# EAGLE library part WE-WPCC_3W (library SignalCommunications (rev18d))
WE-WPCC Wireless Power Charging Coil Characteristics Qi-standard compliant Evaluated and approved by every major semiconductor manufacturer Litzwire used – highest Q-value available on market Applicable for up to 20 W High permeability shielding Cancels charging flux to be not coupled into sensitive components or batteries High reliable construction Applications Portable devices used in a clean area, where connectors pose a risk of polluting e.g. medical facilities, (industrial) clean rooms, mining industry Devices with a large number of mating cycles to avoid connector damage: eg. Smart watches, fitness tracker … Consumer products: eg. Digital cameras, baby phone, walkie talky, remote control, smartphone sleeves, watertight products Explosion sensitive area where the use of a physical connection is hazardous Smart sensors Details see: http://katalog.we-online.de/en/pbs/WE-WPCC-ARRAY Created by Dan Xu 2014-05-21 2014 (C) Wurth Elektronik
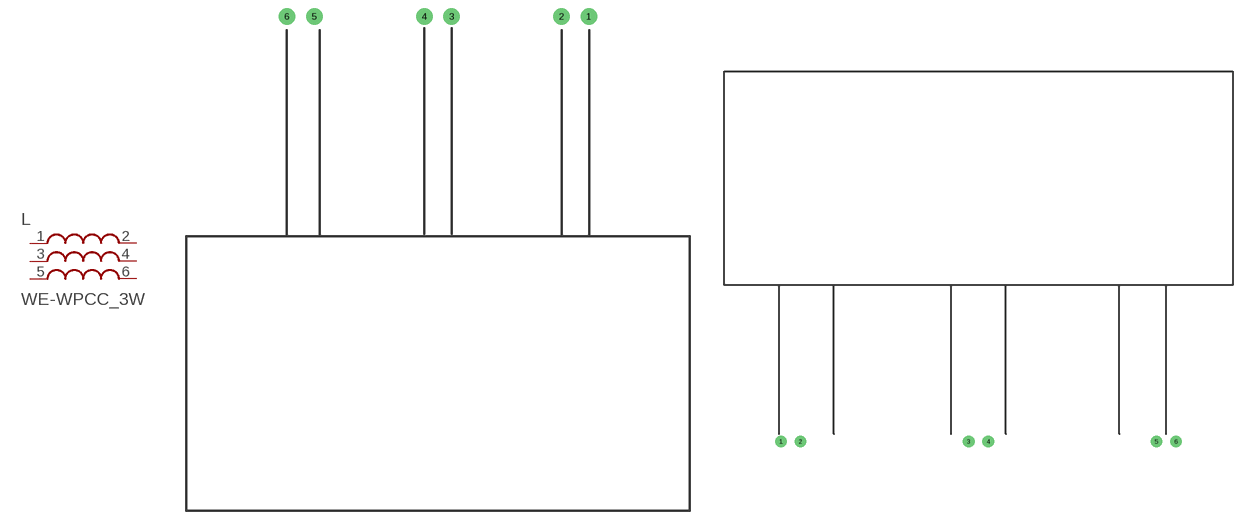
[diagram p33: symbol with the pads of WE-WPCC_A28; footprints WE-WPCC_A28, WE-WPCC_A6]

Designator prefix L

## WE-WPCC_3W_760308104120  [WE-WPCC_A28]
1  1  pas
2  2  pas
3  3  pas
4  4  pas
5  5  pas
6  6  pas

## WE-WPCC_3W_760308106  [WE-WPCC_A6]
Pads as for WE-WPCC_A28

## WE-WPCC_3W_760308103145  [WE-WPCC_MP_A6]
Pads as for WE-WPCC_A28

## WE-WPCC_3W_760308103147  [WE-WPCC_MP_A8]
Pads as for WE-WPCC_A28

## Footprint WE-WPCC_A28 (pad centres in mm)
WE-WPCC Wireless Power Array A28 The distance between two pins is 5.0mm min
drill 2: 1 27.5,0; 2 22.5,0; 3 2.5,0; 4 -2.5,0; 5 -22.5,0; 6 -27.5,0

## Footprint WE-WPCC_A6 (pad centres in mm)
WE-WPCC Wireless Power Array A6 The distance between two pins is 5.0mm min
drill 2: 1 -50.5,0; 2 -45.5,0; 3 -2.5,0; 4 2.5,0; 5 45.5,0; 6 50.5,0

## Footprint WE-WPCC_MP_A6 (pad centres in mm)
drill 2: 1 0,26.57; 2 0,21.57; 3 0,1.43; 4 0,-3.57; 5 0,-19.43; 6 0,-24.43

## Footprint WE-WPCC_MP_A8 (pad centres in mm)
drill 2: 1 0,28.5; 2 0,23.5; 3 0,2.5; 4 0,-2.5; 5 0,-23.5; 6 0,-28.5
